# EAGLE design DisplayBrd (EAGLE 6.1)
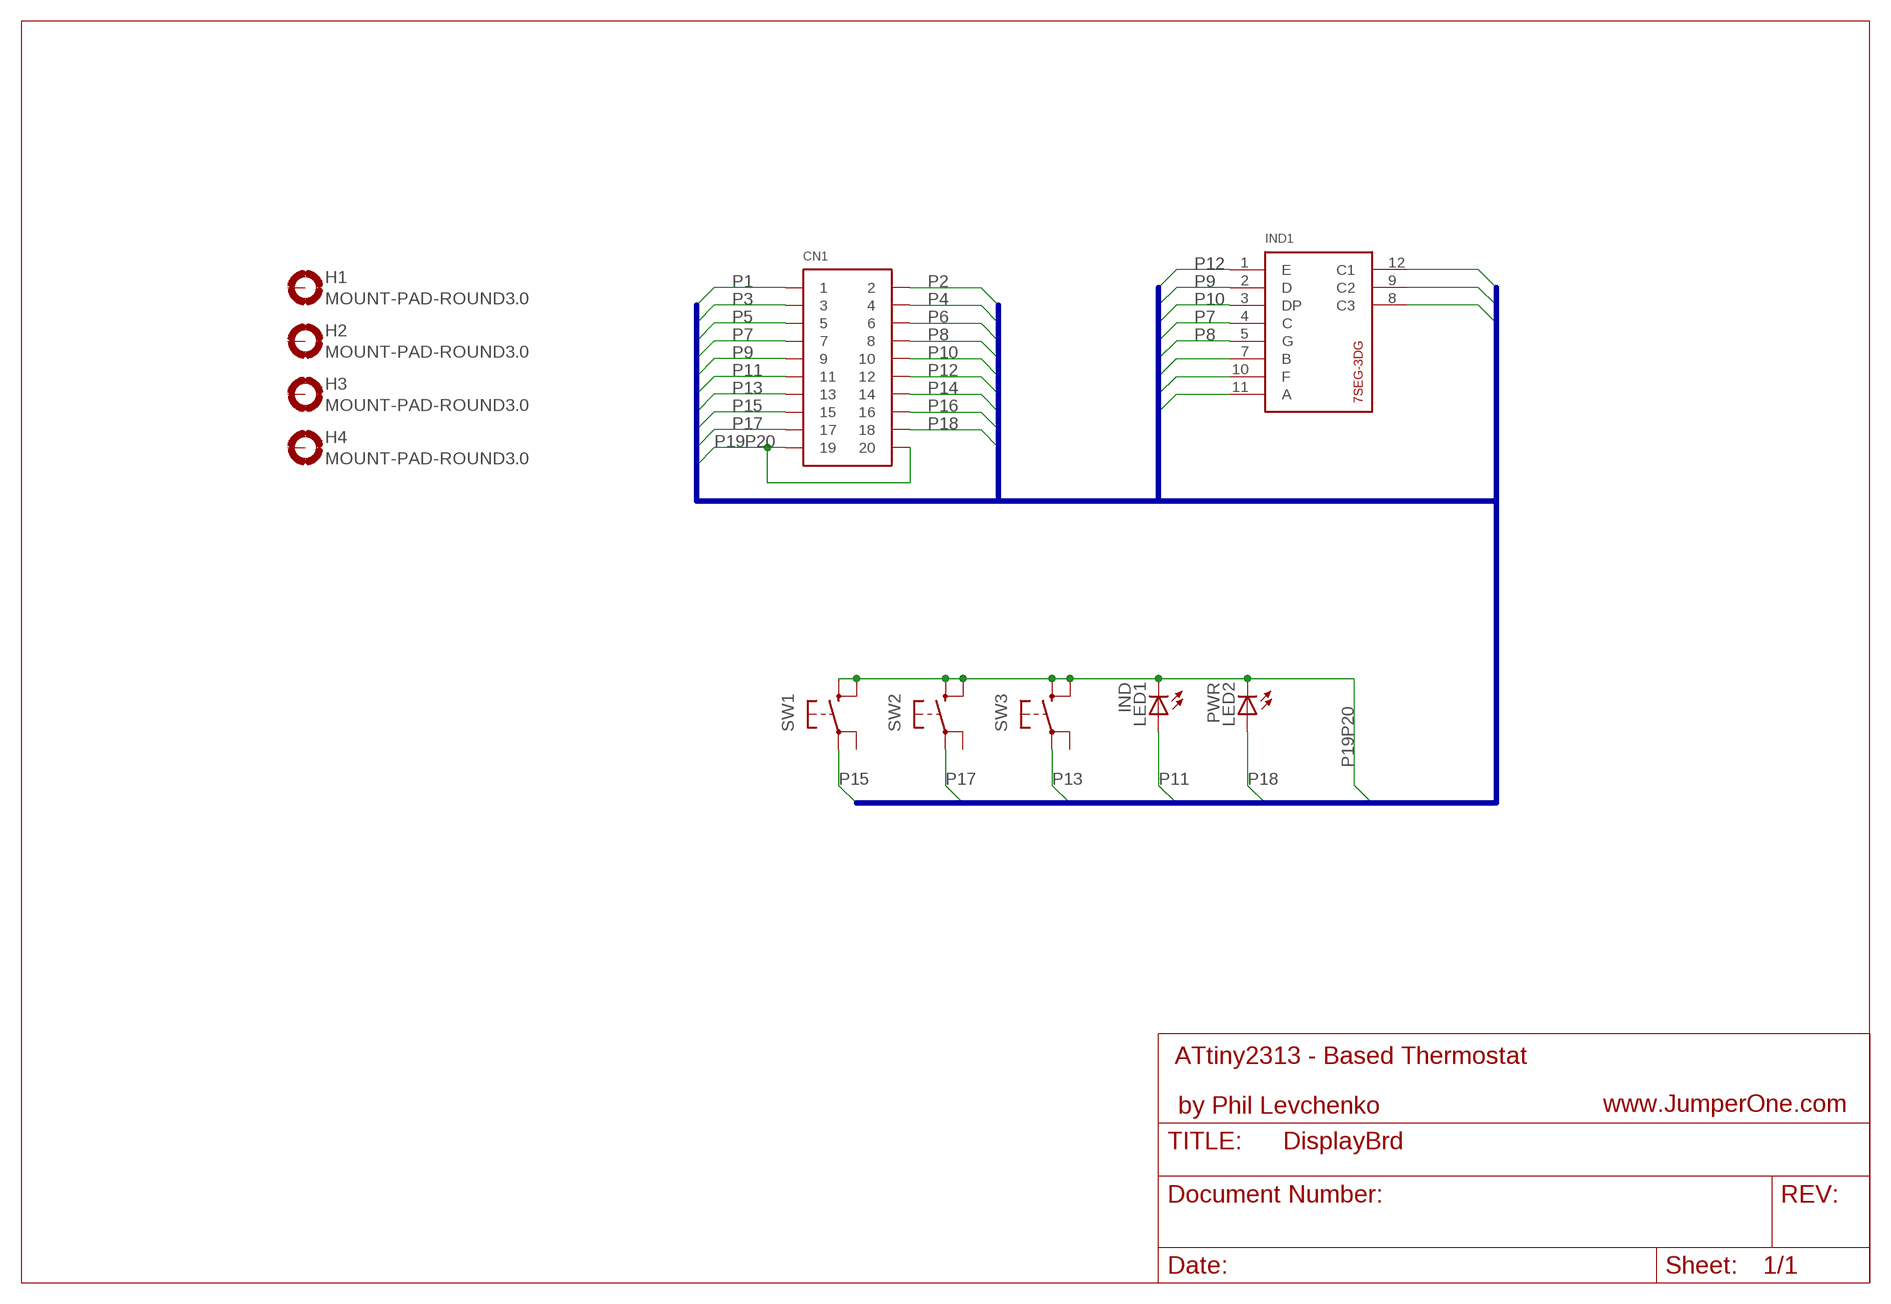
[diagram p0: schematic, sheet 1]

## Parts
CN1  CON-2X10-PH-SMD  [CON-PH-SMD-2X10]
H1  MOUNT-PAD-ROUND3.0  [3,0-PAD]
H2  MOUNT-PAD-ROUND3.0  [3,0-PAD]
H3  MOUNT-PAD-ROUND3.0  [3,0-PAD]
H4  MOUNT-PAD-ROUND3.0  [3,0-PAD]
IND1  7SEG-E30361-L  [7SEG-E30361]
LED1  IND  LED3MM  [LED3MM]
LED2  PWR  LED3MM  [LED3MM]
SW1  SWITCH-TACT-9MM-PCAP  [SWITCH-TACT-9MM]
SW2  SWITCH-TACT-9MM-PCAP  [SWITCH-TACT-9MM]
SW3  SWITCH-TACT-9MM-PCAP  [SWITCH-TACT-9MM]

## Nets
P1: CN1.1 IND1.11(A)
P2: CN1.2 IND1.12(C1)
P3: CN1.3 IND1.10(F)
P4: CN1.4 IND1.9(C2)
P5: CN1.5 IND1.7(B)
P6: CN1.6 IND1.8(C3)
P7: CN1.7 IND1.4(C)
P8: CN1.8 IND1.5(G)
P9: CN1.9 IND1.2(D)
P10: CN1.10 IND1.3(DP)
P11: CN1.11 LED1.A
P12: CN1.12 IND1.1(E)
P13: CN1.13 SW3.1.0(P)
P14: CN1.14
P15: CN1.15 SW1.1.0(P)
P16: CN1.16
P17: CN1.17 SW2.1.0(P)
P18: CN1.18 LED2.A
P19P20: CN1.19 CN1.20 LED1.K(C) LED2.K(C) SW1.2.0(S) SW1.2.1(S1) SW2.2.0(S) SW2.2.1(S1) SW3.2.0(S) SW3.2.1(S1)
Unconnected: H1.B3,0(MOUNT) H2.B3,0(MOUNT) H3.B3,0(MOUNT) H4.B3,0(MOUNT) SW1.1.1(P1) SW2.1.1(P1) SW3.1.1(P1)

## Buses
P[1..20]

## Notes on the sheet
- ATtiny2313 - Based Thermostat
- by Phil Levchenko | www.JumperOne.com

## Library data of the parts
CN1 = JumperOne:CON-2X10
H1-H4 = holes:MOUNT-PAD-ROUND: MOUNTING PAD, round
IND1 = JumperOne:7SEG-E30361-L
LED1 LED2 = JumperOne:LED
SW1-SW3 = JumperOne:SWITCH-TACT

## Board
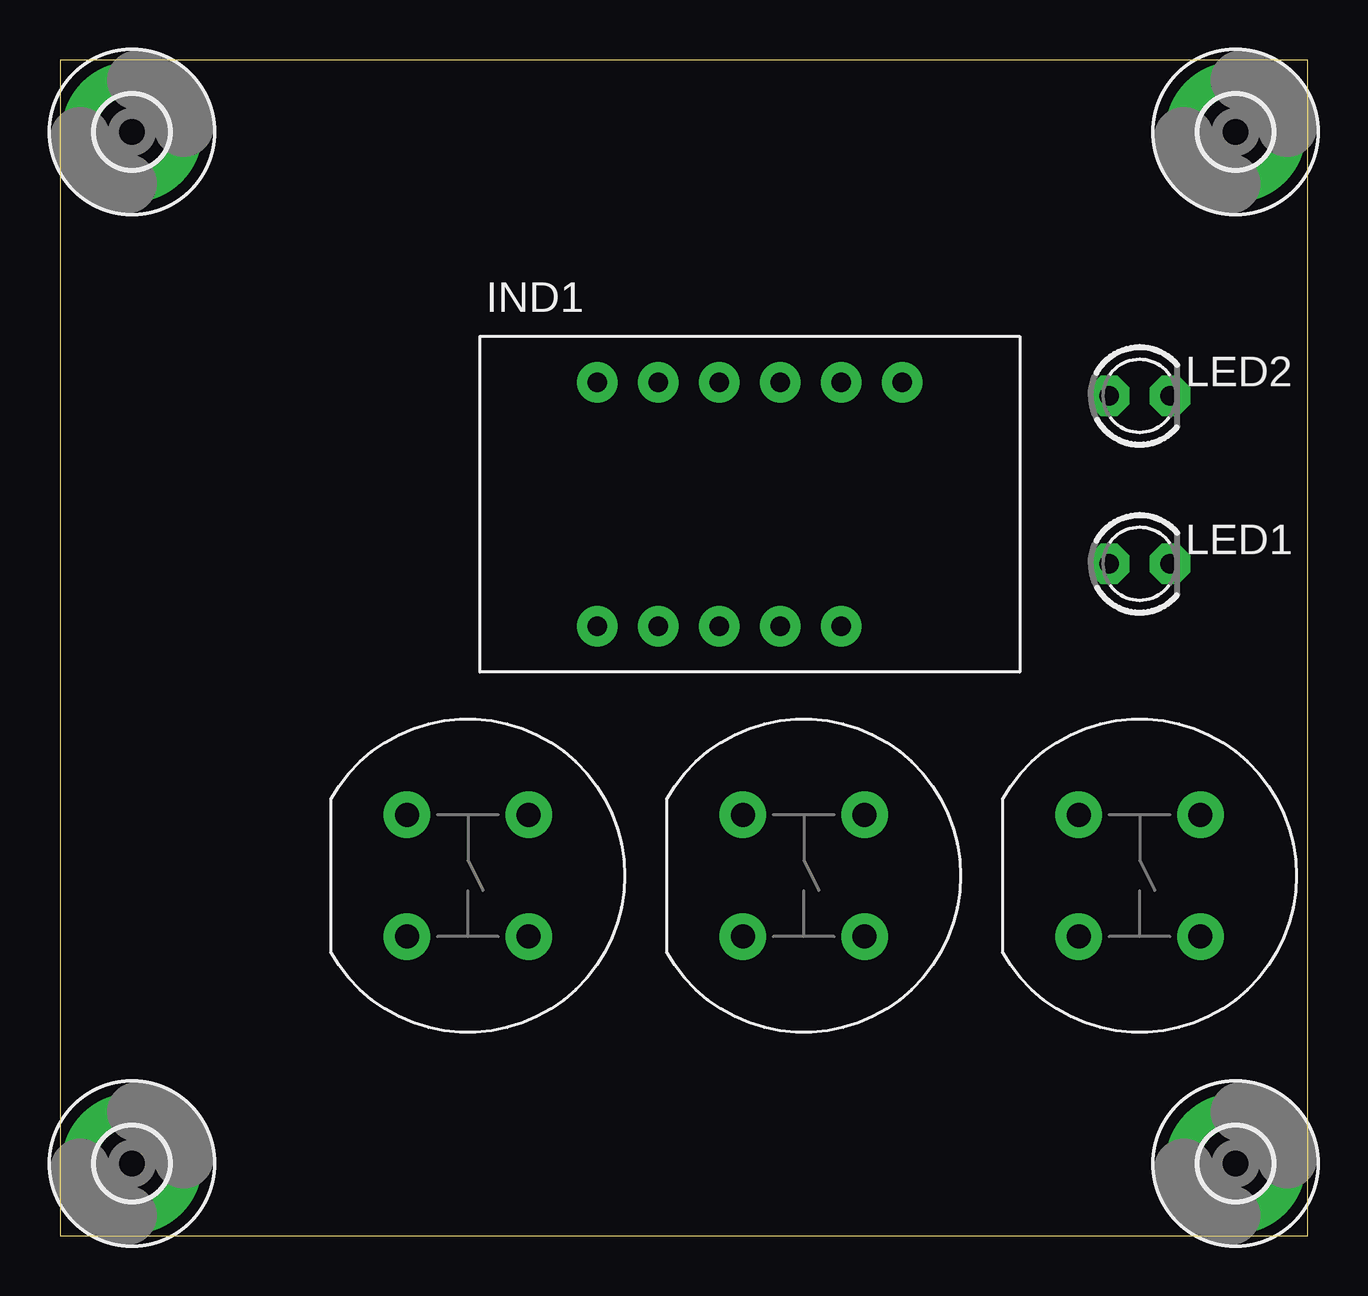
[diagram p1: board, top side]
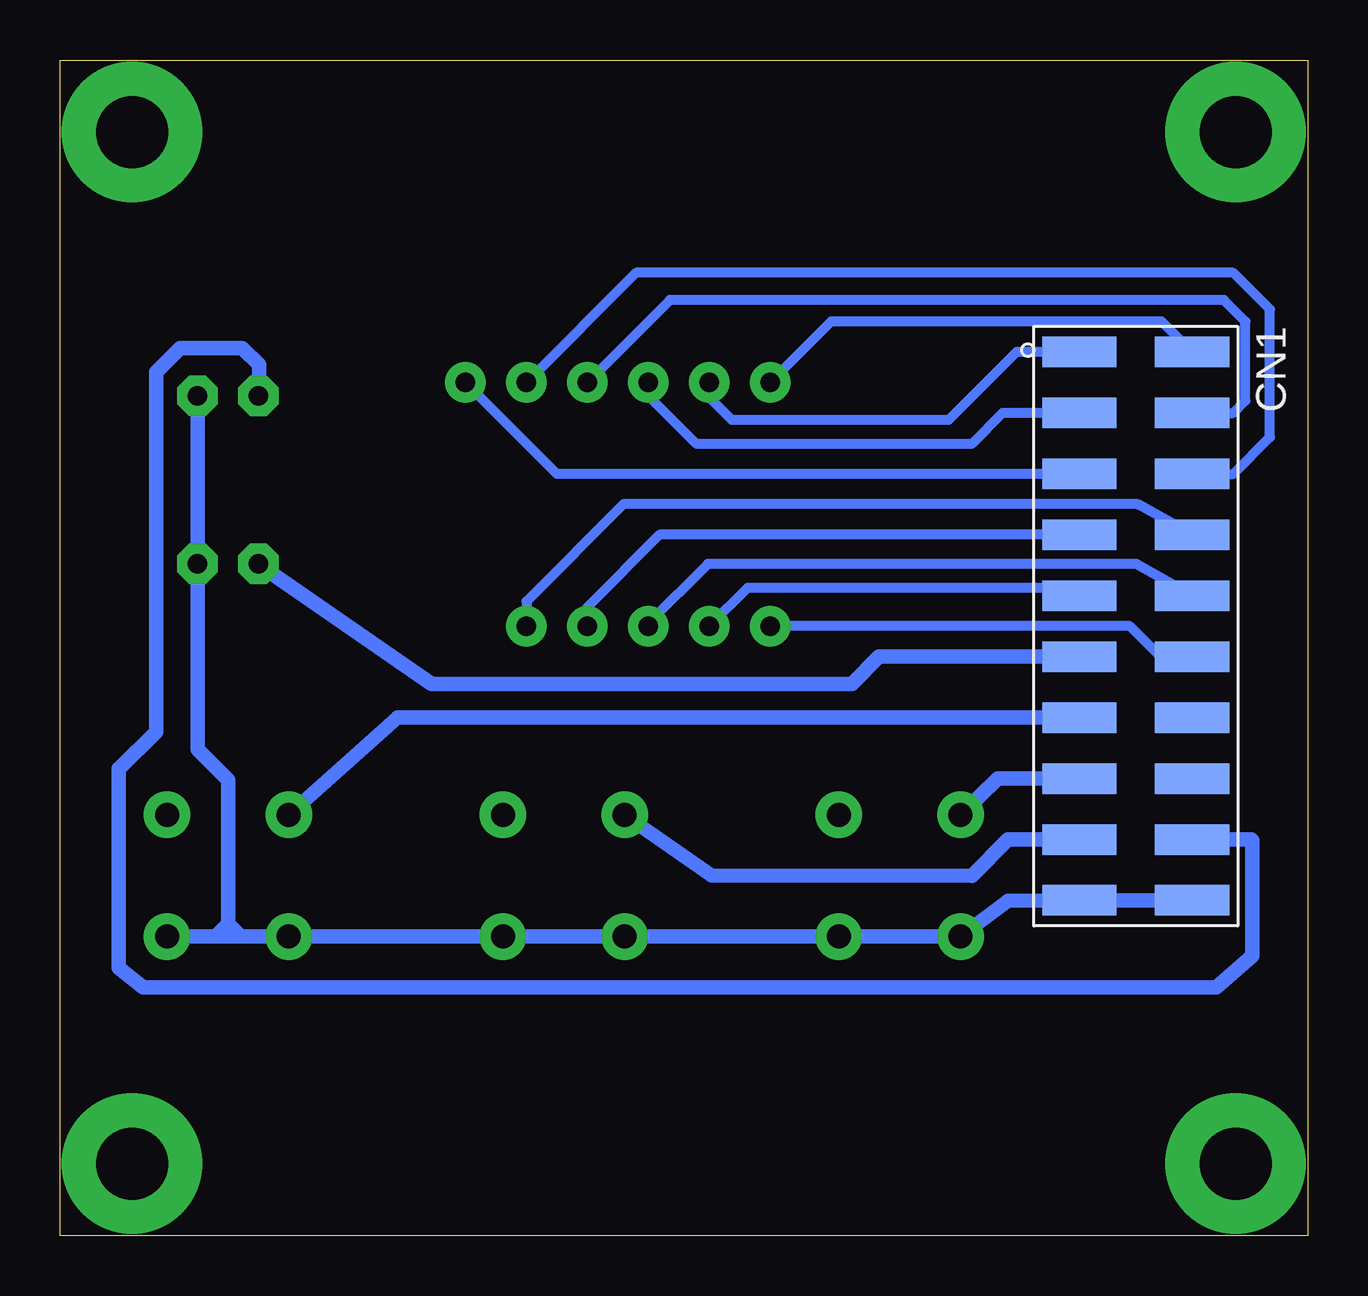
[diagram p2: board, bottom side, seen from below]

Size 52 x 49 mm. Coordinates in mm from the lower left corner, seen from the top.
Outline: 0,0 52,0 52,49 0,49 0,0
Copper layers (1*16): Top 0.035mm / dielectric 1.5mm / Bottom 0.035mm
Design rules: minimum track width 10mil, minimum drill 24mil, track to track 8mil, track to pad 8mil, pad to pad 8mil, via to via 8mil, smd to smd 8mil, copper to edge 40mil, drill to drill 8mil, minimum pad ring 10mil, minimum via ring 8mil, stop-mask expansion 4mil, vias tented up to drill 0mil, thermal gap 10mil

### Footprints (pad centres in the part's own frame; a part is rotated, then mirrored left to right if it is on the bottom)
CON-PH-SMD-2X10 = smd 1.27 x 3.1: 1 -11.43,-2.35; 2 -11.43,2.35; 3 -8.89,-2.35; 4 -8.89,2.35; 5 -6.35,-2.35; 6 -6.35,2.35; 7 -3.81,-2.35; 8 -3.81,2.35; 9 -1.27,-2.35; 10 -1.27,2.35; 11 1.27,-2.35; 12 1.27,2.35; 13 3.81,-2.35; 14 3.81,2.35; 15 6.35,-2.35; 16 6.35,2.35; 17 8.89,-2.35; 18 8.89,2.35; 19 11.43,-2.35; 20 11.43,2.35
3,0-PAD = drill 3 pad 5.842: B3,0 0,0
7SEG-E30361 = drill 0.8 pad 1.676: 1 -6.35,-5.08; 2 -3.81,-5.08; 3 -1.27,-5.08; 4 1.27,-5.08; 5 3.81,-5.08; 7 6.35,5.08; 8 3.81,5.08; 9 1.27,5.08; 10 -1.27,5.08; 11 -3.81,5.08; 12 -6.35,5.08
LED3MM = drill 0.813 pad 1.676 octagon: A -1.27,0; K 1.27,0
SWITCH-TACT-9MM = drill 1 pad 1.93: 1.0 -2.54,-2.54; 1.1 -2.54,2.54; 2.0 2.54,-2.54; 2.1 2.54,2.54

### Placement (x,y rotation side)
CN1  7.16,25.4 270 bottom
H1  49,46 0 top
H2  3,46 0 top
H3  49,3 0 top
H4  3,3 0 top
IND1  28.75,30.48 0 top
LED1  45,28 0 top
LED2  45,35 0 top
SW1  17,15 270 top
SW2  31,15 270 top
SW3  45,15 270 top

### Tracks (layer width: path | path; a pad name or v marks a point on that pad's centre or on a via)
P1
  Bottom 0.406: CN1.1 12.13,36.83 14.96,34 24,34 24.94,34.94 IND1.11
P2
  Bottom 0.406: CN1.2 6.08,38.1 19.86,38.1 IND1.12
P3
  Bottom 0.406: CN1.3 12.71,34.29 14,33 25.46,33 27.48,35.02 IND1.10
P4
  Bottom 0.406: CN1.4 3.1,34.29 2.59,34.8 2.59,38.1 3.49,39 26.58,39 IND1.9
P5
  Bottom 0.406: CN1.5 31.29,31.75 IND1.7
P6
  Bottom 0.406: CN1.6 3.1,31.75 1.57,33.27 1.57,38.61 3.1,40.13 27.99,40.13 IND1.8
P7
  Bottom 0.406: IND1.4 30.02,26.19 27,29.21 CN1.7
P8
  Bottom 0.406: IND1.5 32.56,26.43 28.51,30.48 7.08,30.48 CN1.8
P9
  Bottom 0.406: IND1.2 23.34,27 10,27 9.67,26.67 CN1.9
P10
  Bottom 0.406: IND1.3 27.48,25.52 25,28 7.14,28 CN1.10
P11
  Bottom 0.61: LED1.A 36.51,23 19,23 17.87,24.13 CN1.11
P12
  Bottom 0.406: IND1.1 7.41,25.4 6.14,24.13 CN1.12
P13
  Bottom 0.61: SW3.1.0 37.92,21.59 CN1.13
P15
  Bottom 0.61: SW1.1.0 12.9,19.05 CN1.15
P17
  Bottom 0.61: SW2.1.0 24.85,15.01 14,15 12.49,16.51 CN1.17
P18
  Bottom 0.61: CN1.18 2.35,16.51 2.3,16.46 2.3,11.65 3.81,10.34 48.53,10.34 49.55,11.16 49.55,19.47 49.53,19.47 48,21 48,36 47,37 44.4,37 43.7,36.3 43.7,35.03 LED2.A
P19P20
  Bottom 0.61: 44.46,12.46 45,12.46 | 45,12.46 SW3.2.1 | LED2.K LED1.K 46.27,20.27 45,19 45,13 | CN1.20 CN1.19 12.49,13.95 SW1.2.0 SW1.2.1 SW2.2.0 SW2.2.1 SW3.2.0 44.46,12.46 | 45,12.46 45,13 | 44.46,12.46 45,13 | 45,13 45.5,12.5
